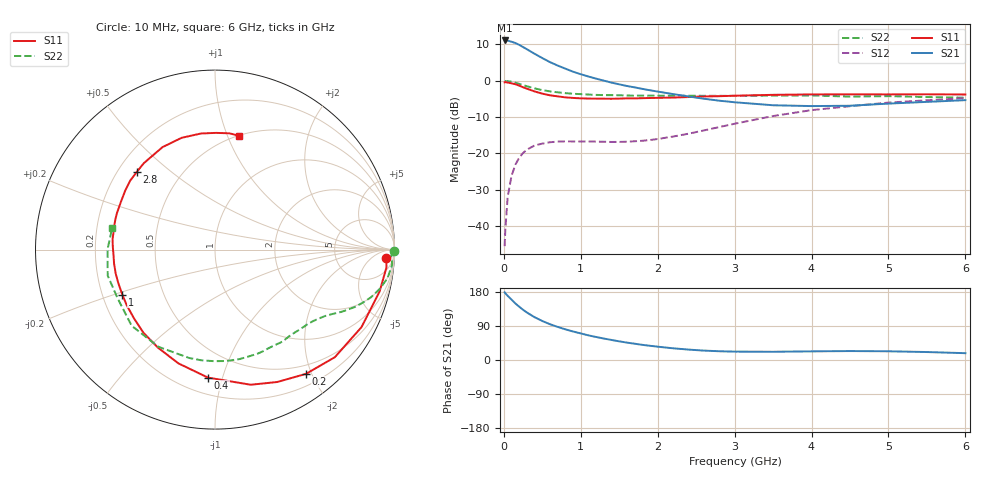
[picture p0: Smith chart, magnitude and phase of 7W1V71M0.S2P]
! Infineon Technologies  Discrete & RF Semiconductors
! BFS17W
! Si NPN RF Bipolar Junction Transistor in SOT323
! VCE = 1.75 V  IC = 1 mA
! Common Emitter S-Parameters:  August  1999
# GHz  S  MA  R  50
!  f  S11  S21  S12  S22
! GHz  MAG  ANG  MAG  ANG  MAG  ANG  MAG  ANG
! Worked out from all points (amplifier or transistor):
!   36 points, 10 MHz to 6 GHz, reference 50 ohm
!   highest |S21| = 11.1 dB at 10 MHz (marker M1)
!   |S21| within 3 dB of that: start of sweep to 346.2 MHz
!   unconditionally stable (mu >= 1): 991.9 MHz to end of sweep
!   at 250 MHz: K = 0.27, MSG = 14.6 dB, |S12| = -19.9 dB
!   at 1.4 GHz: K = 1.32, MAG = 4.8 dB, |S12| = -16.8 dB
!   at 6 GHz: K = 1.12, MAG = -2.3 dB, |S12| = -4.8 dB
!   S11 on the Smith chart (normalised r, x): 10 MHz: 21, -22; 200 MHz: 0.36, -1.92; 400 MHz: 0.31, -0.90; 1 GHz: 0.28, -0.21; 2.8 GHz: 0.28, +0.39; 6 GHz: 0.51, +1.10
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0.01  0.955 -2.7  3.594 178.7  0.0053 88.6  0.9999 -0.5
0.02  0.9605 -5.9  3.59 175.9  0.0092 90.2  0.9827 -1.9
0.05  0.9462 -14.3  3.573 169.3  0.0254 82.5  0.9906 -4.8
0.1  0.9235 -27.9  3.452 159.4  0.0493 74.2  0.9739 -9.5
0.15  0.8974 -41.9  3.313 149.3  0.0701 66.1  0.9417 -13.6
0.2  0.8581 -53.8  3.125 140.5  0.0875 59.9  0.9086 -17.0
0.25  0.8152 -64.8  2.916 132.5  0.1017 53.6  0.8731 -19.9
0.3  0.7788 -75.2  2.719 125.3  0.1131 49.2  0.8426 -22.3
0.4  0.7144 -93.1  2.355 112.9  0.1288 41.4  0.7869 -26.1
0.5  0.666 -107.8  2.056 102.9  0.1367 35.9  0.7453 -28.8
0.6  0.632 -120.2  1.808 94.4  0.1428 32.5  0.7154 -31.2
0.8  0.5918 -139.8  1.47 80.9  0.1468 28.4  0.6763 -36.1
1  0.5741 -154.1  1.232 70.1  0.1463 27.2  0.6559 -40.8
1.1  0.5701 -161.0  1.146 65.0  0.1464 27.3  0.6476 -43.7
1.6  0.5736 174.2  0.849 45.9  0.1452 34.5  0.6277 -58.1
2.2  0.588 153.0  0.657 30.9  0.171 49.0  0.6252 -77.2
2.8  0.6145 135.0  0.533 23.1  0.2308 56.4  0.6213 -97.2
3.5  0.6415 117.1  0.461 21.7  0.3275 54.9  0.6266 -120.2
4  0.65 106.6  0.449 22.8  0.395 49.5  0.629 -137.6
4.5  0.6516 96.8  0.454 23.6  0.4472 43.3  0.6067 -153.2
5.5  0.6528 83.0  0.513 21.0  0.5398 31.1  0.5985 179.8
6  0.6481 77.9  0.542 18.0  0.5758 25.4  0.5856 167.9
